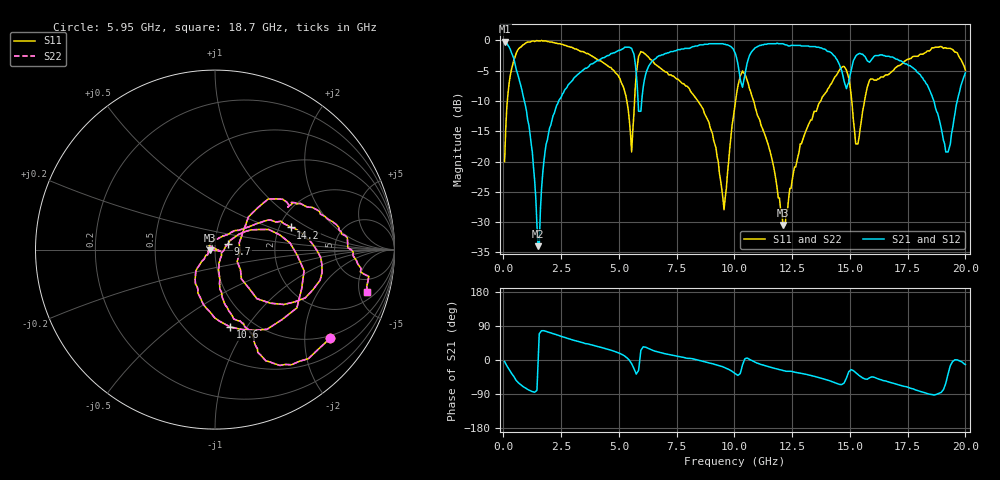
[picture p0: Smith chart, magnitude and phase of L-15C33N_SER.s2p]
# MHZ S MA R 50
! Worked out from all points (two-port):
!   400 points, 50 MHz to 20 GHz, reference 50 ohm
!   highest |S21| = -0.18 dB at 50 MHz (marker M1); lowest = -34.0 dB at 1.5 GHz (marker M2)
!   |S21| within 3 dB of the highest: 6.519 GHz to 10.11 GHz (3.592 GHz wide, 43.2 % of centre); 10.59 GHz to 14.44 GHz (3.846 GHz wide, 30.7 % of centre)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
!   lowest |S11| = -30.5 dB at 12.1 GHz (marker M3), VSWR 1.06, Z = 47.1 - j0.32 ohm
!   |S11| at or under -10 dB: 8.419 GHz to 10.05 GHz (1.628 GHz wide, 17.6 % of centre); 10.83 GHz to 13.73 GHz (2.897 GHz wide, 23.6 % of centre); 15.08 GHz to 15.63 GHz (553.5 MHz wide, 3.6 % of centre)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
!   |S22| runs from -30.5 to 0.0 dB; largest |S21 - S12| = 0
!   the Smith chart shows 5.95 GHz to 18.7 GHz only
!   S11 on the Smith chart (normalised r, x): 5.95 GHz: 0.92, -2.65; 9.7 GHz: 1.16, +0.07; 10.6 GHz: 0.79, -0.84; 14.2 GHz: 2.31, +0.71; 18.7 GHz: 2.88, -6.00
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50  0.1 78.2  0.98 -4.0  0.98 -4.0  0.1 78.2
450  0.69 43.1  0.71 -43.4  0.71 -43.4  0.69 43.1
1150  0.97 7.0  0.17 -80.9  0.17 -80.9  0.97 7.0
1500  0.99 -3.7  0.02 -5.5  0.02 -5.5  0.99 -3.7
2000  0.97 -16.7  0.19 72.6  0.19 72.6  0.97 -16.7
3400  0.81 -45.0  0.56 46.1  0.56 46.1  0.81 -45.0
5050  0.48 -82.6  0.83 17.2  0.83 17.2  0.48 -82.6
5550  0.12 -51.8  0.86 -9.8  0.86 -9.8  0.12 -51.8
5950  0.81 -37.6  0.26 25.5  0.26 25.5  0.81 -37.6
6700  0.61 -67.1  0.74 21.0  0.74 21.0  0.61 -67.1
9700  0.08 23.5  0.92 -23.2  0.92 -23.2  0.08 23.5
10050  0.32 20.5  0.77 -36.5  0.77 -36.5  0.32 20.5
10600  0.44 -78.8  0.7 3.6  0.7 3.6  0.44 -78.8
12100  0.03 -173.5  0.94 -27.6  0.94 -27.6  0.03 -173.5
13350  0.22 34.3  0.89 -41.4  0.89 -41.4  0.22 34.3
14200  0.44 16.3  0.79 -56.5  0.79 -56.5  0.44 16.3
14850  0.57 -28.2  0.4 -47.6  0.4 -47.6  0.57 -28.2
15350  0.14 15.4  0.77 -38.7  0.77 -38.7  0.14 15.4
16700  0.53 28.9  0.74 -58.4  0.74 -58.4  0.53 28.9
18700  0.88 -15.5  0.28 -91.6  0.28 -91.6  0.88 -15.5
19250  0.86 -35.0  0.12 -36.6  0.12 -36.6  0.86 -35.0
20000  0.57 -62.8  0.54 -12.3  0.54 -12.3  0.57 -62.8
